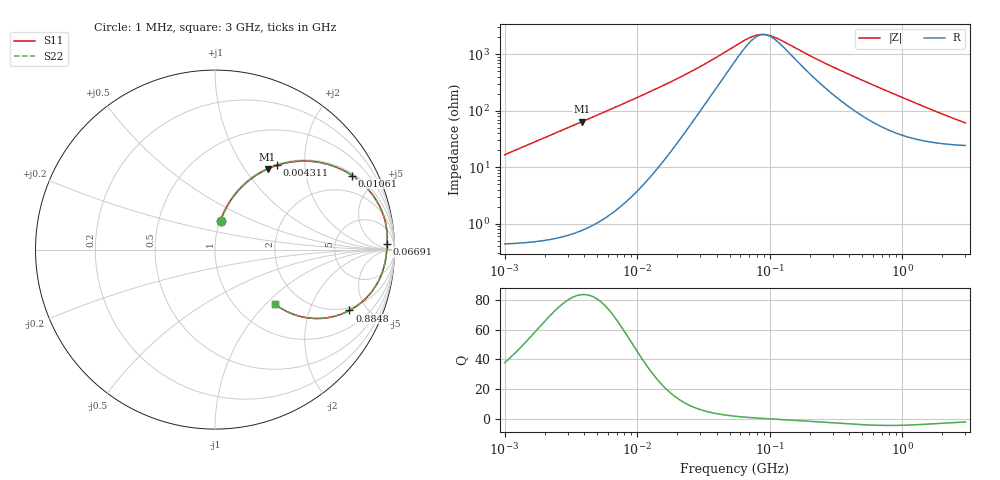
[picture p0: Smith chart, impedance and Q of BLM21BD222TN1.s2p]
! BLM21BD222TN1
# Hz S RI R 50
!Freq.(Hz) S11(Real) S11(Imag) S21(Real) S21(Imag) S12(Real) S12(Imag) S22(Real) S22(Imag)
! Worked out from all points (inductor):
!   401 points, 1 MHz to 3 GHz, reference 50 ohm
!   read as one part in series: L = 2.65 uH near 1.041 MHz
!   highest Q = 83.7 at 3.823 MHz (marker M1), where L = 2.66 uH
!   self-resonance near 91.41 MHz
!   S11 on the Smith chart (normalised r, x): 1 MHz: 1.01, +0.33; 4.311 MHz: 1.02, +1.45; 10.61 MHz: 1.09, +3.65; 66.91 MHz: 29, +24; 884.8 MHz: 1.82, -3.81; 3 GHz: 1.49, -1.12
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1000000  0.0311 0.1608  0.9689 -0.1608  0.9689 -0.1608  0.0311 0.1608
2097170  0.1127 0.309  0.8873 -0.309  0.8873 -0.309  0.1127 0.309
2831560  0.186 0.3828  0.814 -0.3828  0.814 -0.3828  0.186 0.3828
3823119  0.2929 0.4492  0.7071 -0.4492  0.7071 -0.4492  0.2929 0.4492
4310966  0.3449 0.4694  0.6551 -0.4694  0.6551 -0.4694  0.3449 0.4694
6696013  0.5605 0.4891  0.4395 -0.4891  0.4395 -0.4891  0.5605 0.4891
1.061086e7  0.7642 0.4127  0.2358 -0.4127  0.2358 -0.4127  0.7642 0.4127
1.461624e7  0.8602 0.3275  0.1398 -0.3275  0.1398 -0.3275  0.8602 0.3275
2.509235e7  0.9395 0.1879  0.0605 -0.1879  0.0605 -0.1879  0.9395 0.1879
5.477226e7  0.9598 0.0554  0.0402 -0.0554  0.0402 -0.0554  0.9598 0.0554
6.690963e7  0.9592 0.0322  0.0408 -0.0322  0.0408 -0.0322  0.9592 0.0322
8.173662e7  0.958 0.0112  0.042 -0.0112  0.042 -0.0112  0.958 0.0112
9.984923e7  0.9564 -0.00875  0.0436 0.00875  0.0436 0.00875  0.9564 -0.00875
1.195584e8  0.9545 -0.0266  0.0455 0.0266  0.0455 0.0266  0.9545 -0.0266
2.094008e8  0.9434 -0.0886  0.0566 0.0886  0.0566 0.0886  0.9434 -0.0886
4.480278e8  0.8916 -0.2085  0.1084 0.2085  0.1084 0.2085  0.8916 -0.2085
8.005644e8  0.7782 -0.322  0.2218 0.322  0.2218 0.322  0.7782 -0.322
8.848309e8  0.749 -0.3392  0.251 0.3392  0.251 0.3392  0.749 -0.3392
1.194682e9  0.6461 -0.3761  0.3539 0.3761  0.3539 0.3761  0.6461 -0.3761
1.581072e9  0.5387 -0.3827  0.4613 0.3827  0.4613 0.3827  0.5387 -0.3827
2.266846e9  0.4098 -0.3494  0.5902 0.3494  0.5902 0.3494  0.4098 -0.3494
3e9  0.3317 -0.3018  0.6683 0.3018  0.6683 0.3018  0.3317 -0.3018
